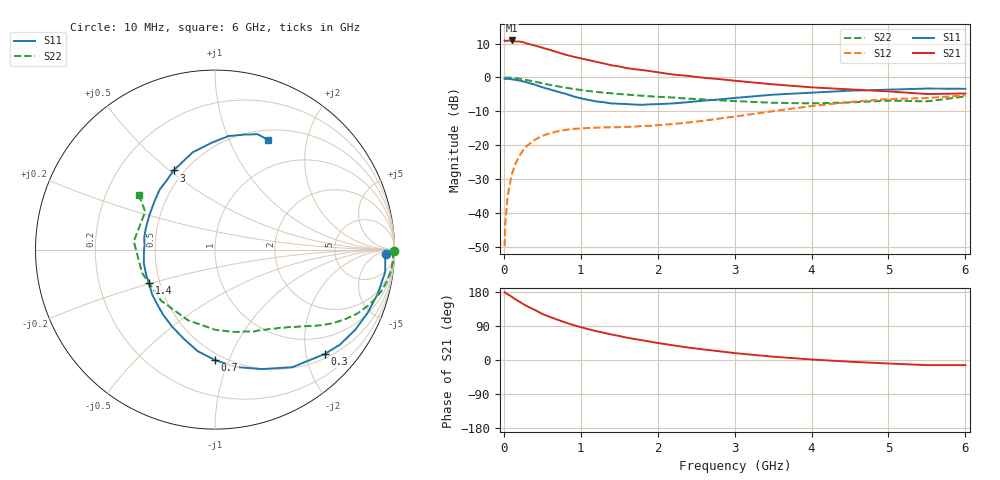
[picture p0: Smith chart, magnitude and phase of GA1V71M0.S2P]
! Infineon Technologies  Discrete & RF Semiconductors
! BF775
! Si NPN RF Bipolar Junction Transistor in SOT23
! VCE = 1.75 V  IC = 1 mA
! Common Emitter S-Parameters:  May  1996
# GHz  S  MA  R  50
!  f  S11  S21  S12  S22
! GHz  MAG  ANG  MAG  ANG  MAG  ANG  MAG  ANG
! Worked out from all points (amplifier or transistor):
!   36 points, 10 MHz to 6 GHz, reference 50 ohm
!   highest |S21| = 10.9 dB at 100 MHz (marker M1)
!   |S21| within 3 dB of that: start of sweep to 629.1 MHz
!   unconditionally stable (mu >= 1): 1.377 GHz to end of sweep
!   at 250 MHz: K = 0.21, MSG = 16.0 dB, |S12| = -21.6 dB
!   at 1.4 GHz: K = 1.02, MAG = 8.4 dB, |S12| = -14.7 dB
!   at 6 GHz: K = 1.06, MAG = -1.2 dB, |S12| = -5.3 dB
!   S11 on the Smith chart (normalised r, x): 10 MHz: 32, -17; 300 MHz: 0.59, -2.38; 700 MHz: 0.45, -0.89; 1.4 GHz: 0.44, -0.20; 3 GHz: 0.44, +0.52; 6 GHz: 0.62, +1.40
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0.01  0.9519 -1.5  3.52 179.1  0.0032 89.9  0.9995 -0.6
0.02  0.9497 -2.9  3.459 177.4  0.0071 85.5  0.9909 -1.3
0.05  0.9564 -7.5  3.497 173.6  0.0178 84.1  0.9942 -3.5
0.1  0.9397 -15.2  3.523 167.3  0.0358 80.8  0.9869 -7.0
0.15  0.9202 -22.6  3.398 160.3  0.0525 75.6  0.9744 -10.4
0.2  0.9001 -29.7  3.4 154.2  0.0686 71.7  0.9585 -13.5
0.25  0.8749 -37.2  3.328 147.9  0.0835 67.0  0.937 -16.7
0.3  0.8437 -43.6  3.171 142.2  0.0971 63.2  0.9139 -19.5
0.4  0.784 -56.7  2.97 132.3  0.1194 56.2  0.8694 -24.2
0.5  0.7151 -68.6  2.751 121.8  0.1367 50.0  0.8193 -28.4
0.7  0.6156 -90.0  2.356 106.1  0.1598 41.2  0.7398 -34.5
0.9  0.5265 -109.3  2.034 92.4  0.1735 35.3  0.6785 -38.9
1.1  0.4647 -128.3  1.809 81.3  0.1789 31.5  0.6301 -43.0
1.4  0.4127 -153.1  1.513 67.3  0.1831 28.9  0.5822 -48.4
1.8  0.394 176.3  1.286 52.1  0.1913 30.2  0.537 -55.4
2.2  0.4126 152.7  1.104 38.8  0.2044 33.2  0.5051 -64.6
3  0.4977 117.6  0.894 18.2  0.2639 37.2  0.4471 -89.7
3.5  0.5562 102.9  0.791 8.8  0.3174 35.3  0.4215 -111.0
4.5  0.637 83.2  0.666 -4.5  0.4342 24.2  0.4265 -162.3
5  0.6597 76.1  0.622 -9.2  0.4791 16.6  0.4548 174.2
5.5  0.6853 69.8  0.569 -13.6  0.4961 8.2  0.4429 151.4
6  0.6791 64.3  0.579 -13.6  0.5427 3.8  0.5233 144.3
